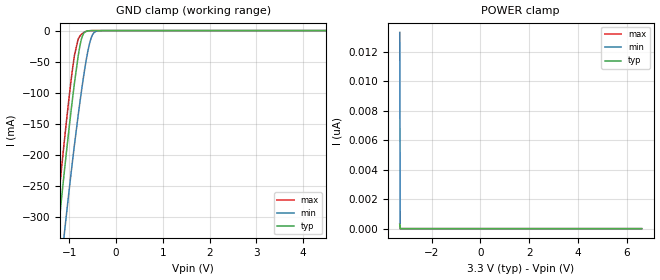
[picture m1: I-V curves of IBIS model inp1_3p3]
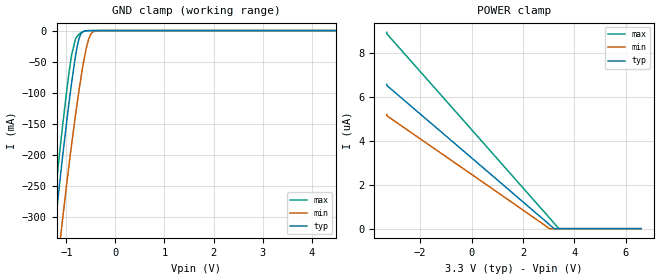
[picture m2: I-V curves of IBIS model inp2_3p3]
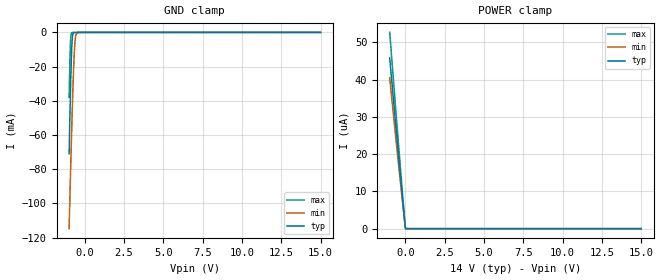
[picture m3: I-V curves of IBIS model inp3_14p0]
|Texas Instruments Incorporated
|TCAN4550 CAN FD Controller with Integrated Transceiver
[IBIS Ver]   4.1
[File name]   tcan4550.ibs
[Date]   03/25/2019
[File Rev]   1.0
[Source]
| Texas Instruments Incorporated.
| Analog-eLab Design Center, HPA
| 12500 TI Blvd
| Dallas, TX -75243
[Notes]   Revision History:
| Rev 1.0: 03/25/2019
| - Initial version of the model
| - Model generated from simulations in SPECTRE
| - Model names with a trailing _3p3 contain the model for 3.3V operation.
|   Model names with a trailing _5p0 contain the model for 5.0V operation.
|   Model names with a trailing _3p6 contain the model for 3.6V operation.
|   Model names with a trailing _6p0 contain the model for 6.0V operation.
|   Model names with a trailing _14p0 contain the model for 14.0V operation.
|   Model names with a trailing _28p0 contain the model for 28.0V operation.
| - C_comp although listed in numerical order of value are
|   obtained from varying PVT conditions. For PVT conditions for
|   each specific value refer the buffer description under
|   respective [Model]. IBIS model user is responsible for using
|   appropriate C_comp to simulate for Signal Integrity.
[Disclaimer]
| This model is designed as an aid for customers of Texas Instruments.
| TI and its licensors and suppliers make no warranties, either expressed
| or implied, with respect to this  model, including the warranties of
| merchantability or fitness for a particular purpose. The model is
| provided solely on an "as is" basis. The entire risk as to its quality
| and performance is with the customer.
| This model is subject to change without notice. Texas Instruments
| Incorporated is not responsible for updating this model.
[Copyright]
(C) Copyright 2019 Texas Instruments Incorporated.All rights reserved.
|  Component TCAN4550RGY 20-Pin VQFN -RGY package
|  Part # TCAN4550RGY
[Component]   TCAN4550RGY
[Manufacturer]  TI
[Package]   |20 VQFN -RGY package
|   typ   min   max
R_pkg   0.05   0.04   0.06
L_pkg   1.0nH   0.8nH   1.2nH
C_pkg   0.2pF   0.16pF   0.24pF
[Pin]  signal_name  model_name  R_pin   L_pin   C_pin
1   OSC1   nc   NA   NA   NA
2   NWKRQ   out_od1   NA   NA   NA
3   GPIO1   i/o   NA   NA   NA
4   SCLK   inp1   NA   NA   NA
5   SDI   inp1   NA   NA   NA
6   SDO   out3   NA   NA   NA
7   NCS   inp1   NA   NA   NA
8   NINT   iood   NA   NA   NA
9   GPO2   out_od2   NA   NA   NA
10   CANL   canl   NA   NA   NA
11   CANH   canh   NA   NA   NA
12   WAKE   inp3   NA   NA   NA
13   GND   gnd   NA   NA   NA
14   VSUP   power   NA   NA   NA
15   INH   os   NA   NA   NA
16   VCCOUT   power   NA   NA   NA
17   VIO   power   NA   NA   NA
18   FLTR   nc   NA   NA   NA
19   RST   inp2   NA   NA   NA
20   OSC2   nc   NA   NA   NA
[Diff Pin]  inv_pin  vdiff  tdelay_typ tdelay_min tdelay_max
10   11   1.15   NA   NA   NA
|   Model Selectors
[Model Selector] inp1
inp1_3p3   3.3V   digital Input
inp1_5p0   5.0V   digital Input
[Model Selector] inp2
inp2_3p3   3.3V   digital Input
inp2_5p0   5.0V   digital Input
[Model Selector] inp3
inp3_6p0   6.0V   digital Input
inp3_14p0   14.0V   digital Input
inp3_28p0   28.0V   digital Input
[Model Selector] i/o
io_3p3   3.3V   digital I/O
io_5p0   5.0V   digital I/O
[Model Selector] out_od1
od1_3p3   3.3V   digital Open-drain
od1_5p0   5.0V   digital Open-drain
out1_3p6   3.6V   digital Output
[Model Selector] out_od2
od2_3p3   3.3V   digital Open-drain
od2_5p0   5.0V   digital Open-drain
out2_3p3   3.3V   digital Output
out2_5p0   5.0V   digital Output
[Model Selector] out3
out3_3p3   3.3V   digital Output
out3_5p0   5.0V   digital Output
[Model Selector] iood
iood_3p3   3.3V   digital Input Open-drain
iood_5p0   5.0V   digital Input Open-drain
[Model Selector] os
os_6p0   6.0V   digital Input
os_14p0   14.0V   digital Input
os_28p0   28.0V   digital Input
| Models and submodels in the file (25): inp1_3p3 (Input), inp1_5p0 (Input), inp2_3p3 (Input), inp2_5p0 (Input), inp3_14p0 (Input), inp3_28p0 (Input), inp3_6p0 (Input), iood_3p3 (I/O_open_drain), iood_5p0 (I/O_open_drain), io_3p3 (I/O), io_5p0 (I/O), od1_3p3 (Open_drain), od1_5p0 (Open_drain), od2_3p3 (Open_drain), od2_5p0 (Open_drain), os_14p0 (Open_source), os_28p0 (Open_source), os_6p0 (Open_source), out1_3p6 (3-state), out2_3p3 (3-state), out2_5p0 (3-state), out3_3p3 (3-state), out3_5p0 (3-state), canh (I/O), canl (I/O)
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|   inp1_3p3 Model
[Model]   inp1_3p3
Model_type   Input
Vinl = 0.99
Vinh = 2.31
|   typ   min   max
C_comp   5.101pF   4.871pF   5.244pF
|  Where Nom  PVT is Nominal Process, 3.3V,   27C
|   Fast PVT is Strong Process,  3.465, -40C
|   Slow PVT is Weak Process,   3.135V, 150C
[Model spec]
|subparameter
Vinl   0.99   0.9405   1.0395
Vinh   2.31   2.1945   2.4255
[Voltage Range]   3.3   3.135   3.465
|Junction Temperature
[Temperature Range]   27   150   -40
[Power Clamp Reference]   3.3   3.135   3.465
[GND Clamp Reference]   0   0   0
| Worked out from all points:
|   GND clamp passes 1 mA (typ) near -0.63 V on its own axis
[GND Clamp]
|   Voltage   I(typ)   I(min)   I(max)
-3.3V     -2.027A    -2.049A    -2.029A
-1.31V    -376.8mA   -472.4mA   -330.2mA
-1.241V   -323.6mA   -421.3mA   -275.7mA
-1.112V   -228.7mA   -328.9mA   -179.4mA
-993.3mV  -147.2mA   -247.9mA   -97.71mA
-894.3mV  -85.08mA   -184.7mA   -40.1mA
-815.1mV  -41.82mA   -137.3mA   -13.98mA
-755.7mV  -17.34mA   -104mA     -7.096mA
-646.8mV  -1.376mA   -49.82mA   -1.412mA
-518.1mV  -66.51uA   -8.585mA   -73.66uA
-359.7mV  -12.57uA   -184.7uA   -14.85uA
6.6V      0A         0A         0A
[POWER Clamp]
|   Voltage   I(typ)   I(min)   I(max)
-3.3V     308.5pA    13.32nA    312.3pA
-3.28V    0A         0A         0A
-3.27V    0A         0A         0A
6.6V      0A         0A         0A
|   inp2_3p3 Model
[Model]   inp2_3p3
Model_type   Input
Vinl = 0.99
Vinh = 2.31
|   typ   min   max
C_comp   5.101pF   4.871pF   5.244pF
|  Where Nom  PVT is Nominal Process, 3.3V,   27C
|   Fast PVT is Strong Process,  3.465, -40C
|   Slow PVT is Weak Process,   3.135V, 150C
[Model spec]
|subparameter
Vinl   0.99   0.9405   1.0395
Vinh   2.31   2.1945   2.4255
[Voltage Range]   3.3   3.135   3.465
|Junction Temperature
[Temperature Range]   27   150   -40
[Power Clamp Reference]   3.3   3.135   3.465
[GND Clamp Reference]   0   0   0
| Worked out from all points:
|   GND clamp passes 1 mA (typ) near -0.63 V on its own axis
[GND Clamp]
|   Voltage   I(typ)   I(min)   I(max)
-3.3V     -2.027A    -2.049A    -2.029A
-1.31V    -376.8mA   -472.4mA   -330.2mA
-1.241V   -323.6mA   -421.3mA   -275.7mA
-1.112V   -228.7mA   -328.9mA   -179.4mA
-993.3mV  -147.2mA   -247.9mA   -97.71mA
-894.3mV  -85.08mA   -184.7mA   -40.1mA
-815.1mV  -41.82mA   -137.3mA   -13.98mA
-755.7mV  -17.34mA   -104mA     -7.09mA
-646.8mV  -1.368mA   -49.82mA   -1.402mA
-518.1mV  -54.69uA   -8.582mA   -59.38uA
-359.7mV  -778.2nA   -175.3uA   -601.1nA
6.6V      0A         0A         0A
[POWER Clamp]
|   Voltage   I(typ)   I(min)   I(max)
-3.3V     6.584uA    5.203uA    8.94uA
-3.29V    6.516uA    5.139uA    8.869uA
3.026V    192.3nA    6.562nA    504.2nA
3.214V    140pA      0A         252.5nA
3.392V    0A         0A         13.28nA
6.6V      0A         0A         0A
|   inp3_14p0 Model
[Model]   inp3_14p0
Model_type   Input
Vinl = 11
Vinh = 12
|   typ   min   max
C_comp   2.498pF   2.430pF   2.533pF
|  Where Nom  PVT is Nominal Process, 14V,   27C
|   Fast PVT is Strong Process,  16V, -40C
|   Slow PVT is Weak Process,   12V, 150C
[Model spec]
|subparameter
Vinl   11   9   13
Vinh   12   10   14
[Voltage Range]   14   12   16
|Junction Temperature
[Temperature Range]   27   150   -40
[Power Clamp Reference]   14   12   16
[GND Clamp Reference]   0   0   0
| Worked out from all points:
|   GND clamp passes 1 mA (typ) near -0.76 V on its own axis
[GND Clamp]
|   Voltage   I(typ)   I(min)   I(max)
-1V       -71.04mA   -114.8mA   -38.01mA
-952mV    -50.42mA   -97.49mA   -17.7mA
-920mV    -37.39mA   -86.12mA   -7.806mA
-904mV    -31.26mA   -80.51mA   -4.56mA
-856mV    -15.3mA    -64.04mA   -626.7uA
-808mV    -5.014mA   -48.34mA   -103.5uA
-776mV    -1.857mA   -38.49mA   -55.86uA
-712mV    -211.6uA   -21.08mA   -40.45uA
-648mV    -47uA      -8.487mA   -36.4uA
-584mV    -29.59uA   -2.267mA   -32.89uA
-504mV    -24.5uA    -313uA     -28.56uA
15V       0A         0A         0A
[POWER Clamp]
|   Voltage   I(typ)   I(min)   I(max)
-1V       45.82uA    40.45uA    52.66uA
-600mV    27.06uA    23.82uA    31.08uA
-200mV    8.725uA    7.71uA     10uA
-8mV      273.3nA    237.2nA    326.5nA
24mV      0A         0A         0A
15V       0A         0A         0A
